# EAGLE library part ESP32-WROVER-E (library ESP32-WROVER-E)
Module: IoT; Bluetooth Low Energy,WiFi; PCB; SMD; 18x31.4x3.3mm Source: Datasheet
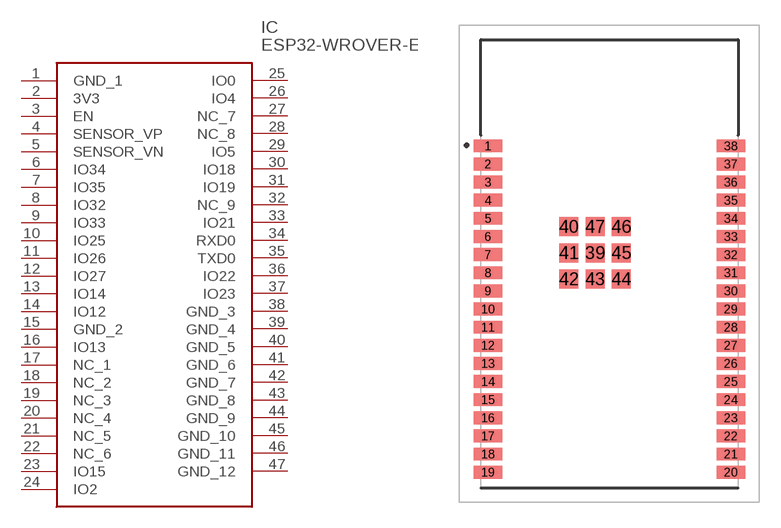
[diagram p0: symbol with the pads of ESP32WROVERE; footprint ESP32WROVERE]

Designator prefix IC

## ESP32-WROVER-E (Description: Module: IoT; Bluetooth Low Energy,WiFi; PCB; SMD; 18x31.4x3.3mm; Height: 3.45mm; Manufacturer_Name: Espressif Systems; Manufacturer_Part_Number: ESP32-WROVER-E)  [ESP32WROVERE]
1  GND_1
2  3V3
3  EN
4  SENSOR_VP
5  SENSOR_VN
6  IO34
7  IO35
8  IO32
9  IO33
10  IO25
11  IO26
12  IO27
13  IO14
14  IO12
15  GND_2
16  IO13
17  NC_1
18  NC_2
19  NC_3
20  NC_4
21  NC_5
22  NC_6
23  IO15
24  IO2
25  IO0
26  IO4
27  NC_7
28  NC_8
29  IO5
30  IO18
31  IO19
32  NC_9
33  IO21
34  RXD0
35  TXD0
36  IO22
37  IO23
38  GND_3
39  GND_4
40  GND_5
41  GND_6
42  GND_7
43  GND_8
44  GND_9
45  GND_10
46  GND_11
47  GND_12

## Footprint ESP32WROVERE (pad centres in mm)
ESP32-WROVER-E-2
smd 2 x 0.9: 1 -7.5,7.5; 2 -7.5,6.23; 3 -7.5,4.96; 4 -7.5,3.69; 5 -7.5,2.42; 6 -7.5,1.15; 7 -7.5,-0.12; 8 -7.5,-1.39; 9 -7.5,-2.66; 10 -7.5,-3.93; 11 -7.5,-5.2; 12 -7.5,-6.47; 13 -7.5,-7.74; 14 -7.5,-9.01; 15 -7.5,-10.28; 16 -7.5,-11.55; 17 -7.5,-12.82; 18 -7.5,-14.09; 19 -7.5,-15.36; 20 9.5,-15.36; 21 9.5,-14.09; 22 9.5,-12.82; 23 9.5,-11.55; 24 9.5,-10.28; 25 9.5,-9.01; 26 9.5,-7.74; 27 9.5,-6.47; 28 9.5,-5.2; 29 9.5,-3.93; 30 9.5,-2.66; 31 9.5,-1.39; 32 9.5,-0.12; 33 9.5,1.15; 34 9.5,2.42; 35 9.5,3.69; 36 9.5,4.96; 37 9.5,6.23; 38 9.5,7.5
smd 1.33 x 1.33: 39 0,0; 40 -1.835,1.835; 41 -1.835,0; 42 -1.835,-1.835; 43 0,-1.835; 44 1.835,-1.835; 45 1.835,0; 46 1.835,1.835; 47 0,1.835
